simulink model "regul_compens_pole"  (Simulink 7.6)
settings: Solver=ode45  StartTime=0.0  StopTime=10.0  RelTol=1e-3
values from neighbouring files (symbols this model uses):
  k = 1000    [masse_ressort_enveloppe.m]
undefined symbols (not defined in the file or in its folder): tau
libraries: fl_lib x4

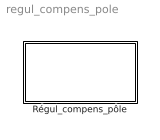
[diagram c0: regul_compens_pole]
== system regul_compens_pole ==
  Régul_compens_pôle : Subsystem

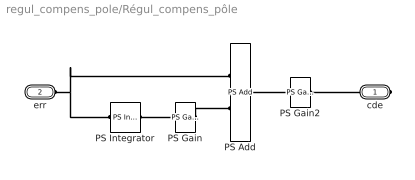
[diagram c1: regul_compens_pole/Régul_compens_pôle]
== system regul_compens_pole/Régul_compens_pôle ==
  PS Add : fl_lib/Physical Signals/Functions/PS Add  DialogController=NetworkEngine.DynNeDlgSource  SystemSampleTime=-1  LocalVarLogging=[]
  PS Gain : fl_lib/Physical Signals/Functions/PS Gain  DialogController=NetworkEngine.DynNeDlgSource  SystemSampleTime=-1  gain=1/tau  LocalVarLogging=[]
  PS Gain2 : fl_lib/Physical Signals/Functions/PS Gain  DialogController=NetworkEngine.DynNeDlgSource  SystemSampleTime=-1  gain=k  LocalVarLogging=[]
  PS Integrator : fl_lib/Physical Signals/Linear Operators/PS Integrator  DialogController=NetworkEngine.DynNeDlgSource  SystemSampleTime=-1  x0=0  x_Log=off  LocalVarNames=|x  LocalVarDescs=|x  LocalVarLogging=0
  cde : PMIOPort  Port=1  Side=Right
  err : PMIOPort  Port=2  Side=Left
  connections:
  err/RConn1 -- PS Integrator/LConn1 -- PS Add/LConn1
  PS Gain/RConn1 -- PS Add/LConn2
  PS Integrator/RConn1 -- PS Gain/LConn1
  PS Gain2/RConn1 -- cde/RConn1
  PS Add/RConn1 -- PS Gain2/LConn1
